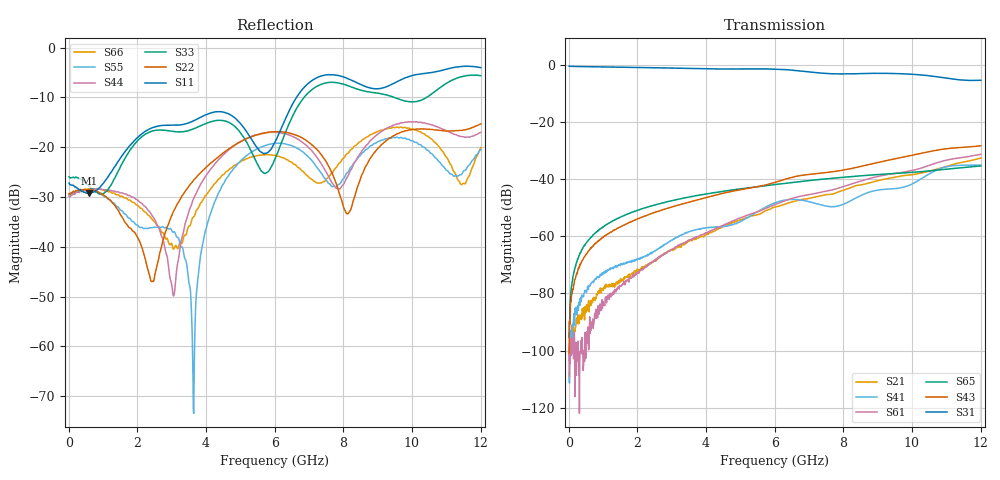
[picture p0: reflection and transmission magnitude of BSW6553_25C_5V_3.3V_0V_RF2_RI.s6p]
! Agilent Technologies	N5230C	MY49001333	A.09.33.09
!	Test time	=	2026-05-26	 10:00
!	Product	=	BSW6553
!	Temp	=	25C
!	Logic	=	RF2
!	Port1	=	RFC
!	Port2	=	RF1
!	Port3	=	RF2
!	Port4	=	RF3
!	Port5	=	RF4
!	Port6	=	RF5
!S6P File: Measurements: <S11,S12,S13,S14,S15,S16>,
!<S21,S22,S23,S24,S25,S26>,
!<S31,S32,S33,S34,S35,S36>,
!<S41,S42,S43,S44,S45,S46>,
!<S51,S52,S53,S54,S55,S56>,
!<S61,S62,S63,S64,S65,S66>;
# HZ S RI R 50
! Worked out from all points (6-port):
!   1201 points, 10 MHz to 12.01 GHz, reference 50 ohm
!   strongest paths, dB at 10 MHz, 3.01 GHz, 6.01 GHz, 9.01 GHz, 12.01 GHz:
!     S31: -0.5, -1.2, -1.5, -3.0, -5.4
!     S43: -100.9, -49.7, -41.2, -34.2, -28.4
!     S65: -95.4, -47.6, -41.9, -38.4, -35.4
!     S61: -98.7, -64.6, -48.9, -39.1, -31.3
!     S41: -108.0, -61.4, -48.3, -43.9, -35.1
!     S21: -103.3, -65.0, -49.8, -40.6, -32.7
!   lowest |S11| = -29.3 dB at 580 MHz (marker M1), VSWR 1.07, Z = 49.8 - j3.43 ohm
!   |S11| at or under -10 dB: start of sweep to 6.638 GHz
